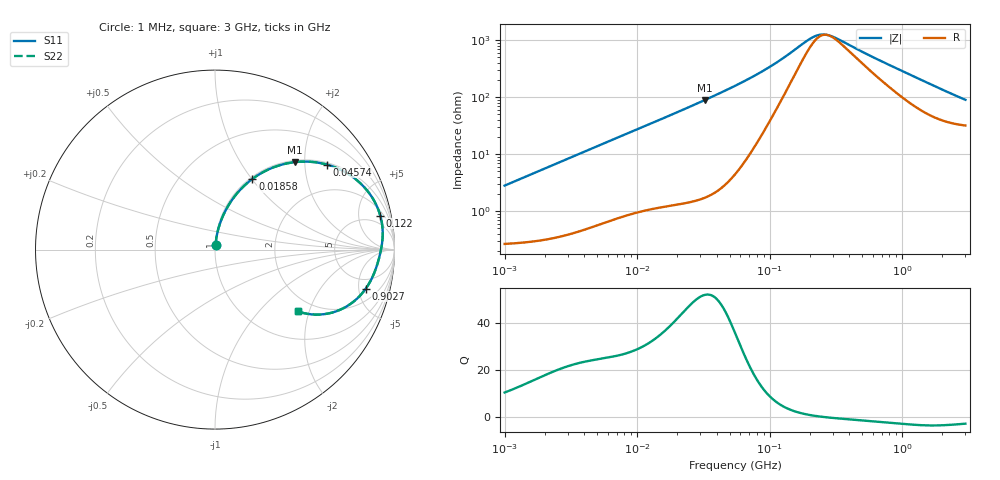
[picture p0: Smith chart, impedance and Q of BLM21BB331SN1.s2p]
! BLM21BB331SN1
# Hz S RI R 50
!Freq.(Hz) S11(Real) S11(Imag) S21(Real) S21(Imag) S12(Real) S12(Imag) S22(Real) S22(Imag)
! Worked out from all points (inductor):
!   401 points, 1 MHz to 3 GHz, reference 50 ohm
!   read as one part in series: L = 445 nH near 1.041 MHz
!   highest Q = 51.7 at 32.55 MHz (marker M1), where L = 437 nH
!   self-resonance near 272.2 MHz
!   S11 on the Smith chart (normalised r, x): 1 MHz: 1.01, +0.06; 18.58 MHz: 1.03, +1.01; 45.74 MHz: 1.06, +2.58; 122 MHz: 2.74, +8.97; 902.7 MHz: 3.39, -5.97; 3 GHz: 1.64, -1.68
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1000000  0.00344 0.0278  0.9966 -0.0278  0.9966 -0.0278  0.00344 0.0278
2097170  0.00659 0.058  0.9934 -0.058  0.9934 -0.058  0.00659 0.058
3823119  0.0156 0.1041  0.9844 -0.1041  0.9844 -0.1041  0.0156 0.1041
8345207  0.0567 0.2135  0.9433 -0.2135  0.9433 -0.2135  0.0567 0.2135
1.461624e7  0.1428 0.3357  0.8572 -0.3357  0.8572 -0.3357  0.1428 0.3357
1.858443e7  0.2082 0.3936  0.7918 -0.3936  0.7918 -0.3936  0.2082 0.3936
2.41077e7  0.3043 0.4494  0.6957 -0.4494  0.6957 -0.4494  0.3043 0.4494
3.254976e7  0.4452 0.4874  0.5548 -0.4874  0.5548 -0.4874  0.4452 0.4874
4.574308e7  0.6215 0.4741  0.3785 -0.4741  0.3785 -0.4741  0.6215 0.4741
5.477226e7  0.7083 0.4408  0.2917 -0.4408  0.2917 -0.4408  0.7083 0.4408
8.173662e7  0.853 0.3226  0.147 -0.3226  0.147 -0.3226  0.853 0.3226
1.219755e8  0.9207 0.19  0.0793 -0.19  0.0793 -0.19  0.9207 0.19
2.094008e8  0.9325 0.0502  0.0675 -0.0502  0.0675 -0.0502  0.9325 0.0502
2.457655e8  0.9283 0.0186  0.0717 -0.0186  0.0717 -0.0186  0.9283 0.0186
2.884452e8  0.9229 -0.0102  0.0771 0.0102  0.0771 0.0102  0.9229 -0.0102
5.364635e8  0.8932 -0.1147  0.1068 0.1147  0.1068 0.1147  0.8932 -0.1147
8.005644e8  0.8567 -0.1919  0.1433 0.1919  0.1433 0.1919  0.8567 -0.1919
9.0272e8  0.8401 -0.2175  0.1599 0.2175  0.1599 0.2175  0.8401 -0.2175
1.294266e9  0.7652 -0.2953  0.2348 0.2953  0.2348 0.2953  0.7652 -0.2953
1.818868e9  0.6541 -0.3506  0.3459 0.3506  0.3459 0.3506  0.6541 -0.3506
2.312676e9  0.5598 -0.3622  0.4402 0.3622  0.4402 0.3622  0.5598 -0.3622
3e9  0.4611 -0.3441  0.5389 0.3441  0.5389 0.3441  0.4611 -0.3441
